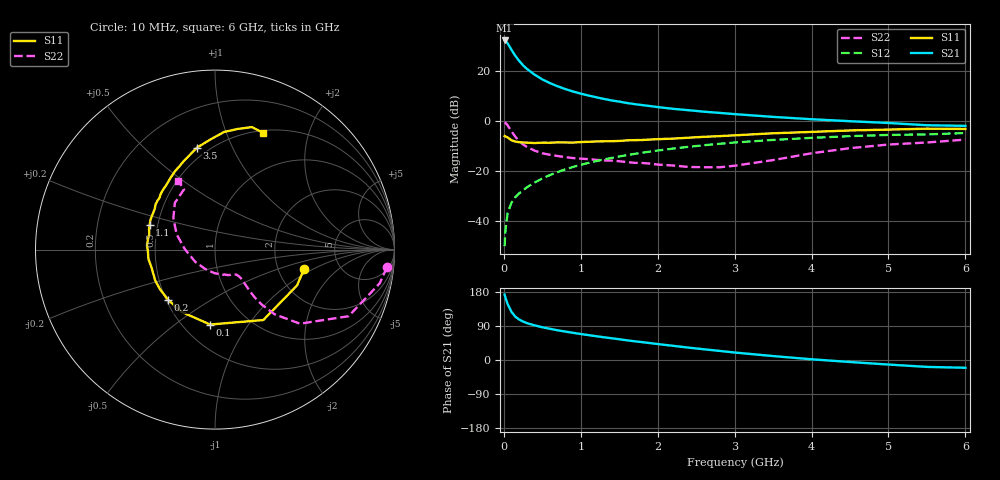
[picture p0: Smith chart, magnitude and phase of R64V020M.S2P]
! SIEMENS Small Signal Semiconductors
! BFR193
! Si NPN RF Bipolar Junction Transistor in SOT23
! VCE = 4 V  IC = 20 mA
! Common Emitter S-Parameters:  May  1996
# GHz  S  MA  R  50
!  f  S11  S21  S12  S22
! GHz  MAG  ANG  MAG  ANG  MAG  ANG  MAG  ANG
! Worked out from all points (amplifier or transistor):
!   36 points, 10 MHz to 6 GHz, reference 50 ohm
!   highest |S21| = 32.3 dB at 10 MHz (marker M1)
!   |S21| within 3 dB of that: start of sweep to 85.32 MHz
!   unconditionally stable (mu >= 1): 572.4 MHz to 1.964 GHz
!   at 250 MHz: K = 0.83, MSG = 25.0 dB, |S12| = -27.5 dB
!   at 1.4 GHz: K = 1.03, MAG = 10.5 dB, |S12| = -14.6 dB
!   at 6 GHz: K = 0.94, MSG = 1.4 dB, |S12| = -4.7 dB
!   lowest NFmin = 1.40 dB at 450 MHz
!   S11 on the Smith chart (normalised r, x): 10 MHz: 2.80, -0.81; 100 MHz: 0.67, -0.68; 200 MHz: 0.51, -0.33; 1.1 GHz: 0.45, +0.15; 3.5 GHz: 0.44, +0.74; 6 GHz: 0.53, +1.36
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0.01  0.5081 -12.1  41.32 172.6  0.0032 83.7  0.963 -5.9
0.02  0.4987 -23.6  40.62 165.5  0.0065 78.8  0.9365 -11.6
0.05  0.4759 -55.5  36.05 147.3  0.015 70.3  0.8317 -26.5
0.1  0.4185 -93.7  26.82 126.8  0.0237 64.5  0.6279 -41.1
0.15  0.3938 -118.2  20.29 114.3  0.0305 62.5  0.4908 -47.3
0.2  0.383 -133.1  16.09 106.7  0.0364 63.3  0.4031 -49.6
0.25  0.3776 -144.3  13.16 101.4  0.042 64.2  0.3452 -50.3
0.3  0.375 -152.6  11.17 97.3  0.048 65.8  0.3087 -50.1
0.4  0.3676 -164.2  8.567 91.4  0.0598 67.3  0.2596 -49.1
0.5  0.3744 -171.9  6.892 86.4  0.072 68.5  0.2298 -48.0
0.6  0.374 -178.7  5.798 82.3  0.0846 68.7  0.2143 -47.9
0.7  0.3798 176.5  5.012 78.3  0.097 68.8  0.2027 -48.1
0.8  0.3781 171.2  4.405 75.0  0.1096 68.3  0.1924 -48.7
0.9  0.3758 166.9  3.939 71.7  0.1226 67.7  0.1844 -49.3
1.1  0.3897 159.3  3.279 65.7  0.1479 66.3  0.1752 -53.1
1.3  0.3986 151.6  2.804 60.0  0.1733 64.1  0.1658 -57.0
1.6  0.416 142.6  2.325 51.9  0.2111 60.7  0.1531 -66.4
2.2  0.4516 126.7  1.779 37.4  0.2852 52.9  0.1309 -91.9
3.5  0.5769 100.0  1.227 10.4  0.4248 33.4  0.1681 179.1
4.5  0.6573 85.6  1.006 -5.3  0.5059 19.1  0.2909 142.9
5.5  0.7131 73.2  0.835 -18.2  0.547 4.8  0.3778 117.1
6  0.7037 67.6  0.811 -20.5  0.584 0.6  0.4315 118.3
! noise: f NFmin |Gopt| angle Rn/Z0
0.45  1.4  0.3  160  0.1
0.9  1.45  0.34  172  0.11
1.8  2.2  0.56  -148  0.2
